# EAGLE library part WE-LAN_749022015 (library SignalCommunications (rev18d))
LAN-Transformer WE-LAN 10/10/1000 Base Tx - Compliant with IEEE 802.3 standards - SMD -- Ethernet -- Power over Ethernet -- 1 Gigabit Ethernet -- Compliant with most IC's for ethernet applications like Intel, AMD, Globespan and Realtek -- Hub, Router, Switch Details see: http://katalog.we-online.de/en/pbs/WE-LAN/S/749022015? Updated by Dan Xu 2014-07-08 2014 (C) Würth Elektronik
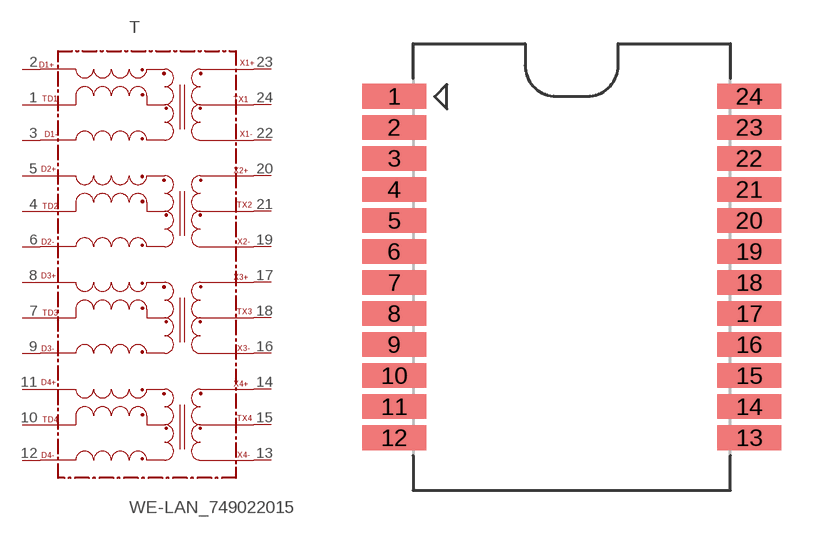
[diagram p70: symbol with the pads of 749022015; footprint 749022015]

Designator prefix T

## WE-LAN_749022015  [749022015]
1  TD1
2  D1+
3  D1-
4  TD2
5  D2+
6  D2-
7  TD3
8  D3+
9  D3-
10  TD4
11  D4+
12  D4-
13  X4-
14  X4+
15  TX4
16  X3-
17  X3+
18  TX3
19  X2-
20  X2+
21  TX2
22  X1-
23  X1+
24  TX1

## Footprint 749022015 (pad centres in mm)
MAX Height = 10.26 mm
smd 2.62 x 1.01: 1 -7.265,6.985; 2 -7.265,5.715; 3 -7.265,4.445; 4 -7.265,3.175; 5 -7.265,1.905; 6 -7.265,0.635; 7 -7.265,-0.635; 8 -7.265,-1.905; 9 -7.265,-3.175; 10 -7.265,-4.445; 11 -7.265,-5.715; 12 -7.265,-6.985; 13 7.265,-6.985; 14 7.265,-5.715; 15 7.265,-4.445; 16 7.265,-3.175; 17 7.265,-1.905; 18 7.265,-0.635; 19 7.265,0.635; 20 7.265,1.905; 21 7.265,3.175; 22 7.265,4.445; 23 7.265,5.715; 24 7.265,6.985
